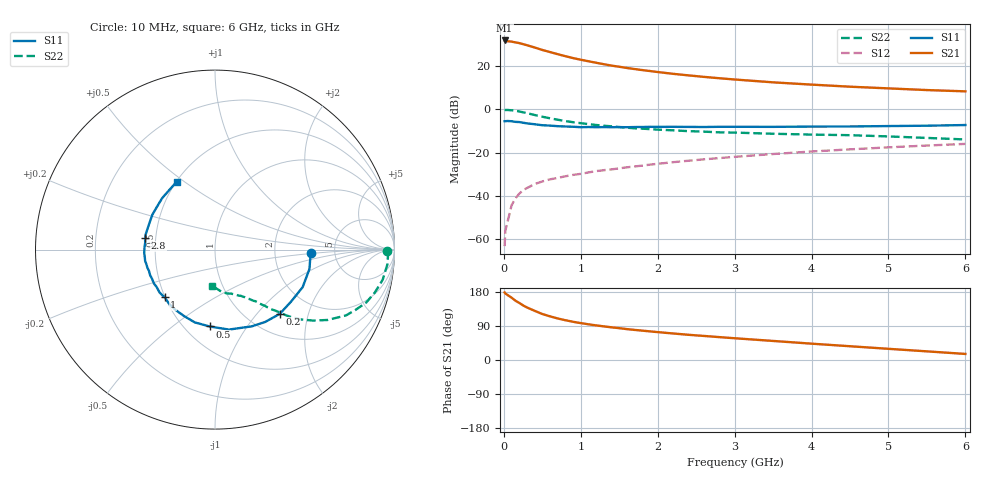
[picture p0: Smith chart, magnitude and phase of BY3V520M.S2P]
! SIEMENS Small Signal Semiconductors
! BFY420
! Si NPN RF SIEGET Grounded Emitter Transistor in MICRO-X
! VCE = 3.5 V  IC = 20 mA
! Common Emitter S-Parameters:  October  1996
# GHz  S  MA  R  50
!  f  S11  S21  S12  S22
! GHz  MAG  ANG  MAG  ANG  MAG  ANG  MAG  ANG
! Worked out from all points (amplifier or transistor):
!   36 points, 10 MHz to 6 GHz, reference 50 ohm
!   highest |S21| = 31.7 dB at 10 MHz (marker M1)
!   |S21| within 3 dB of that: start of sweep to 376.6 MHz
!   unconditionally stable (mu >= 1): start of sweep to 12.29 MHz; 2.003 GHz to end of sweep
!   at 250 MHz: K = 0.31, MSG = 33.7 dB, |S12| = -37.3 dB
!   at 1.4 GHz: K = 0.90, MSG = 23.9 dB, |S12| = -27.7 dB
!   at 6 GHz: K = 1.07, MAG = 10.5 dB, |S12| = -15.9 dB
!   S11 on the Smith chart (normalised r, x): 10 MHz: 3.27, -0.19; 200 MHz: 1.38, -1.33; 500 MHz: 0.66, -0.69; 1 GHz: 0.50, -0.31; 2.8 GHz: 0.44, +0.07; 6 GHz: 0.50, +0.47
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0.01  0.5327 -2.2  38.63 178.2  0.0007 72.3  0.959 -0.5
0.02  0.533 -5.0  38.42 175.4  0.0016 61.7  0.9646 -1.5
0.05  0.5371 -11.7  37.1 171.3  0.0026 77.2  0.9644 -4.8
0.1  0.5313 -23.2  36.3 164.6  0.0061 78.3  0.9493 -10.2
0.15  0.5135 -34.3  34.91 156.6  0.0088 74.4  0.9222 -15.0
0.2  0.5083 -44.8  33.54 150.7  0.0113 72.6  0.8927 -19.3
0.25  0.4907 -55.2  31.77 144.1  0.0137 68.2  0.8523 -23.2
0.3  0.4744 -64.3  30.03 138.7  0.0153 66.7  0.8165 -26.7
0.4  0.4523 -80.1  26.58 129.8  0.0189 63.0  0.7398 -32.0
0.5  0.4294 -93.9  23.35 121.4  0.0217 60.8  0.6745 -35.9
0.6  0.421 -105.5  20.85 115.2  0.0243 60.0  0.6206 -38.9
0.7  0.4084 -115.0  18.67 109.6  0.0262 59.2  0.5749 -41.2
0.9  0.3962 -129.6  15.16 100.8  0.0308 58.1  0.504 -44.1
1  0.387 -136.6  13.88 97.4  0.0325 58.7  0.4789 -45.3
1.1  0.3905 -142.3  12.81 94.2  0.0351 58.9  0.4558 -46.7
1.6  0.3864 -162.0  8.965 81.5  0.046 59.3  0.3767 -51.2
2.2  0.3948 -177.4  6.573 70.0  0.0604 57.6  0.3278 -56.2
2.8  0.3948 170.6  5.205 60.4  0.075 55.1  0.2944 -60.9
3.5  0.3938 158.6  4.184 50.3  0.0931 50.9  0.2732 -66.2
4.5  0.4021 143.2  3.319 36.3  0.1193 43.3  0.2532 -74.8
5.5  0.4186 127.4  2.776 22.8  0.1461 34.6  0.2188 -87.1
6  0.434 119.4  2.593 16.0  0.1595 29.9  0.2018 -95.3
